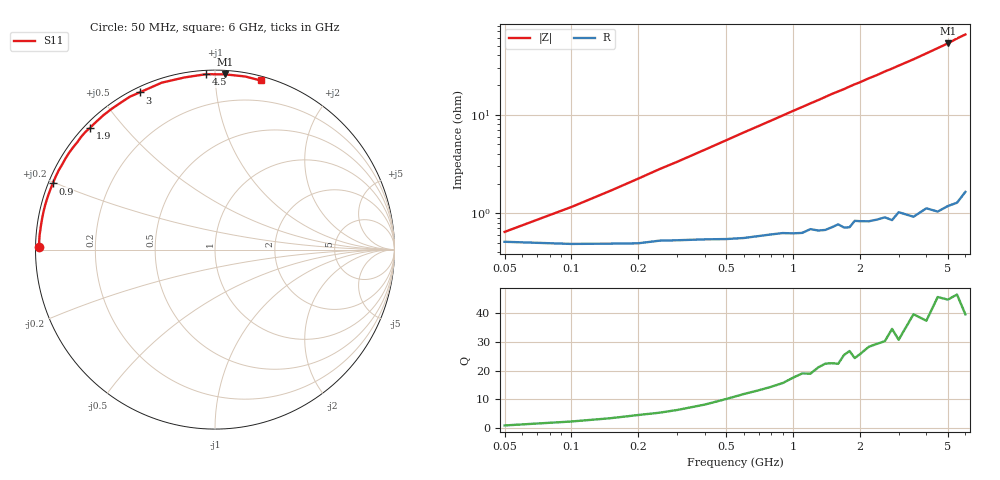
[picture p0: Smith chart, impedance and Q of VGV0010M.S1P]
! Infineon Technologies  Discrete & RF Semiconductors
! BB 831
! Si Tuning Diode in SOD323
! VR =
! S-Parameters:  July  1999
# GHz  S  MA  R  50
!  f  S11
! GHz  MAG  ANG
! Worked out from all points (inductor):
!   34 points, 50 MHz to 6 GHz, reference 50 ohm
!   read as one part to ground: L = 1.74 nH near 150 MHz
!   highest Q = 45.7 at 5 GHz (marker M1), where L = 1.69 nH
!   S11 on the Smith chart (normalised r, x): 50 MHz: 0.01, +0.01; 900 MHz: 0.01, +0.20; 1.9 GHz: 0.02, +0.41; 3 GHz: 0.02, +0.63; 4.5 GHz: 0.02, +0.95; 6 GHz: 0.03, +1.31
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0.05  0.9797 179.1
0.1  0.9807 177.6
0.2  0.9805 175.0
0.4  0.9787 170.0
0.6  0.9782 165.0
0.8  0.9766 160.2
0.9  0.9761 157.8
1  0.9765 155.4
1.1  0.9764 153.1
1.3  0.9756 148.6
1.4  0.9755 146.3
1.5  0.9743 144.0
1.6  0.9728 142.0
1.7  0.975 140.0
1.8  0.9753 137.8
1.9  0.9717 135.7
2  0.9723 133.9
2.2  0.9732 129.8
2.4  0.9729 126.3
2.6  0.9725 122.4
2.8  0.975 119.1
3  0.9711 115.6
3.5  0.9763 107.7
4  0.974 100.0
4.5  0.9784 93.0
5  0.978 86.7
5.5  0.9791 80.1
6  0.9759 74.9
